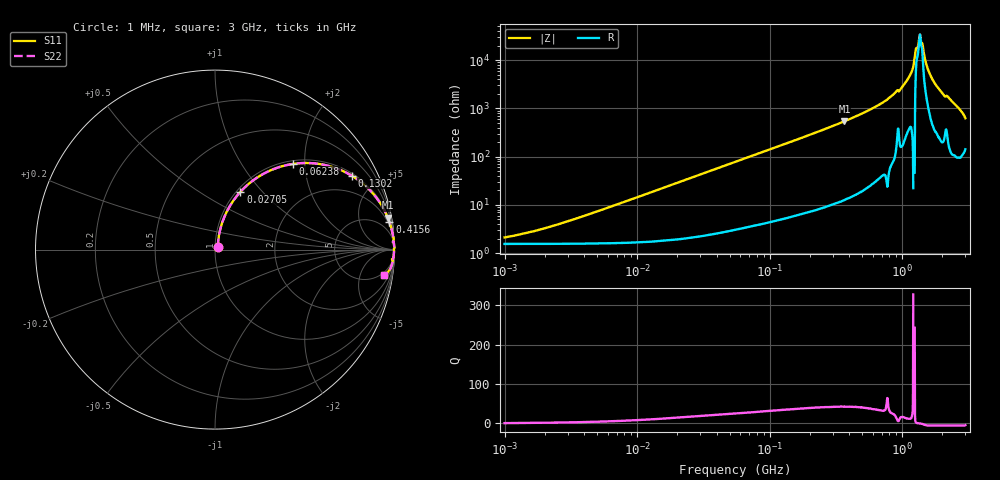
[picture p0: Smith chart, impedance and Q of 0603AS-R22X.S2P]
!s-Parameter Generated by FASTRON Sdn. Bhd.
!FASTRON P/N : 0603AS-R22X
!Keysight Technologies: E4991B_MY54100416_A.01.15
!Date created: Wed Sep 27 15:57:42 2023
!Version  : Rev01 Wed Sep 27 15:57:42 2023
!Data & Calibration Information:
!Freq	S11	S21	S12	S22
!PortZ  Port1:50+j0  Port2:50+j0
!When reading reference impedance value at option line is always used.
! Remarks : This data is being provided solely for informational purposes.
# Hz S dB R 50
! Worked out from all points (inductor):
!   1601 points, 1 MHz to 3 GHz, reference 50 ohm
!   read as one part in series: L = 227 nH near 3.29 MHz
!   highest Q = 42.9 at 366.8 MHz (marker M1), where L = 234 nH
!   self-resonance near 1.361 GHz
!   S11 on the Smith chart (normalised r, x): 1 MHz: 1.03, +0.03; 27.05 MHz: 1.04, +0.77; 62.38 MHz: 1.07, +1.75; 130.2 MHz: 1.10, +3.63; 415.6 MHz: 1, +12; 3 GHz: 4, -12
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1000000  -33.63 42.0  -0.13 -0.8  -0.13 -0.8  -33.63 42.0
3804036  -25.09 70.8  -0.15 -3.1  -0.15 -3.1  -25.09 70.8
1.447069e7  -14.03 73.7  -0.33 -11.4  -0.33 -11.4  -14.03 73.7
2.704826e7  -9.08 66.3  -0.75 -20.5  -0.75 -20.5  -9.08 66.3
5.477226e7  -4.46 51.0  -2.18 -36.7  -2.18 -36.7  -4.46 51.0
6.238265e7  -3.79 47.6  -2.63 -40.3  -2.63 -40.3  -3.79 47.6
1.30174e8  -1.25 28.4  -6.44 -59.9  -6.44 -59.9  -1.25 28.4
2.083556e8  -0.54 18.7  -9.89 -69.9  -9.89 -69.9  -0.54 18.7
3.667557e8  -0.18 10.5  -14.81 -78.2  -14.81 -78.2  -0.18 10.5
4.156301e8  -0.14 9.1  -16.04 -79.6  -16.04 -79.6  -0.14 9.1
7.925923e8  -0.03 3.5  -24.27 -84.9  -24.27 -84.9  -0.03 3.5
9.730857e8  -0.03 2.3  -28.00 -84.1  -28.00 -84.1  -0.03 2.3
1.130699e9  -0.02 1.3  -33.11 -84.0  -33.11 -84.0  -0.02 1.3
1.194682e9  -0.01 0.9  -36.01 -86.7  -36.01 -86.7  -0.01 0.9
1.313842e9  -0.03 0.2  -45.61 -46.1  -45.61 -46.1  -0.03 0.2
1.374365e9  -0.03 -0.1  -49.76 18.6  -49.76 18.6  -0.03 -0.1
1.409185e9  -0.03 -0.2  -46.84 36.0  -46.84 36.0  -0.03 -0.2
1.54974e9  -0.02 -0.8  -36.85 78.6  -36.85 78.6  -0.02 -0.8
1.730092e9  -0.03 -1.6  -31.10 82.2  -31.10 82.2  -0.03 -1.6
2.03054e9  -0.06 -2.9  -25.96 81.4  -25.96 81.4  -0.06 -2.9
2.255531e9  -0.07 -3.5  -24.32 81.0  -24.32 81.0  -0.07 -3.5
3e9  -0.41 -8.6  -16.32 68.3  -16.32 68.3  -0.41 -8.6
